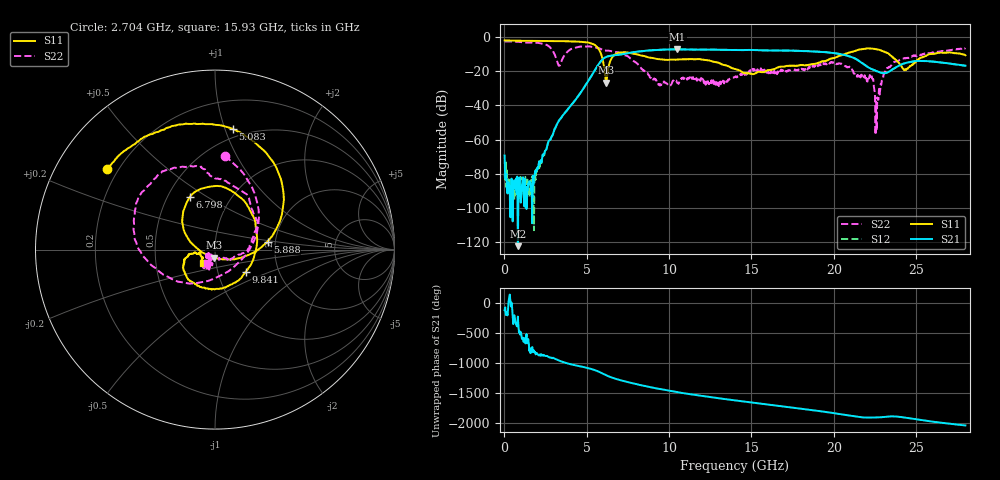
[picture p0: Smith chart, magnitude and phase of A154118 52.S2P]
!  2-Port S-parameters saved by WinCal
! VAR MeasName=S-Parameters (CALIBRATED_DATA) read from VNA (N5230A)
! VAR MeasDate=2015-9-10 14:39:10
! VAR NAME=A154118 52
! VAR FILENAME=A154118 52.S2P
! VAR DATE=2015-9-10 14:39:10
! VAR PHYS_PORTS=1,2
# Hz S DB R 50
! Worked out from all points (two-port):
!   801 points, 10 MHz to 28 GHz, reference 50 ohm
!   highest |S21| = -7.36 dB at 10.51 GHz (marker M1); lowest = -122.2 dB at 814.7 MHz (marker M2)
!   |S21| within 3 dB of the highest: 7.045 GHz to 20.54 GHz (13.5 GHz wide, 97.9 % of centre)
!   lowest |S11| = -26.8 dB at 6.168 GHz (marker M3), VSWR 1.10, Z = 49.3 - j4.48 ohm
!   |S11| at or under -10 dB: 5.866 GHz to 6.766 GHz (899.4 MHz wide, 14.2 % of centre); 7.946 GHz to 20.71 GHz (12.77 GHz wide, 89.1 % of centre); 23.34 GHz to 26.09 GHz (2.751 GHz wide, 11.1 % of centre)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
!   |S22| runs from -57.3 to -2.7 dB; largest |S21 - S12| = 0.0076
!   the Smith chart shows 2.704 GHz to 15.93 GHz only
!   S11 on the Smith chart (normalised r, x): 2.704 GHz: 0.16, +0.32; 5.083 GHz: 0.42, +1.06; 5.888 GHz: 1.82, +0.18; 6.798 GHz: 0.65, +0.42; 9.841 GHz: 1.36, -0.35; 15.93 GHz: 0.87, -0.13
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1e7  -2.15 179.7  -69.31 -126.4  -79.74 -121.3  -2.68 179.8
8.147125e8  -2.29 168.8  -122.22 127.4  -88.44 -135.7  -2.92 159.8
1.82935e9  -2.41 156.0  -81.23 -106.4  -79.57 -123.0  -3.45 134.1
2.704038e9  -2.47 143.3  -60.55 173.8  -60.86 174.8  -5.61 84.0
3.50875e9  -2.60 129.0  -46.34 98.4  -46.42 98.3  -13.17 -120.9
4.698325e9  -3.01 98.2  -31.66 17.3  -31.64 17.1  -5.72 142.4
5.083188e9  -3.35 81.7  -25.92 -8.0  -25.87 -7.8  -5.64 125.1
5.8879e9  -10.57 8.8  -13.93 -86.2  -13.87 -86.2  -7.36 95.6
6.1678e9  -26.83 -95.9  -11.81 -124.1  -11.76 -124.3  -8.10 86.8
6.797575e9  -9.78 115.7  -10.68 171.7  -10.65 171.4  -8.94 63.3
8.057125e9  -10.26 54.6  -8.70 84.6  -8.68 84.4  -15.61 -6.2
9.351662e9  -13.05 -7.7  -7.68 10.6  -7.63 10.4  -27.90 -71.8
9.841488e9  -13.49 -35.5  -7.46 -14.3  -7.43 -14.5  -27.25 -89.5
1.050625e10  -13.25 -73.2  -7.36 -45.8  -7.33 -46.4  -27.06 -107.9
1.4005e10  -18.88 -171.9  -7.74 177.8  -7.71 177.3  -23.52 -112.5
1.592931e10  -19.90 -130.9  -7.99 111.6  -7.89 111.0  -20.97 -121.4
1.869332e10  -15.87 -118.6  -8.53 16.4  -8.53 15.9  -16.73 -107.2
2.226205e10  -6.82 -157.2  -18.67 -106.6  -18.65 -108.1  -22.51 -156.9
2.264691e10  -7.44 -170.3  -20.16 -104.8  -20.13 -106.2  -35.37 62.9
2.334666e10  -10.06 170.0  -20.49 -88.4  -20.47 -89.5  -17.56 -19.2
2.43613e10  -19.14 -167.4  -15.35 -108.6  -15.31 -109.6  -12.61 -61.9
2.8e10  -10.81 177.1  -16.85 122.2  -16.91 121.2  -6.55 -101.9
